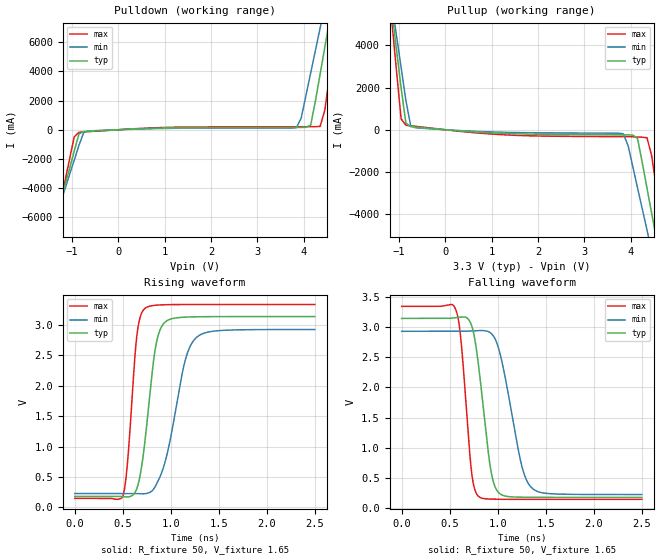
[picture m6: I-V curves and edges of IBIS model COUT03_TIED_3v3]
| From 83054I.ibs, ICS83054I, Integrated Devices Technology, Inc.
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[Model] COUT03_TIED_3v3
Model_type   Output
Polarity   Non-Inverting
|   typ   min   max
C_comp   2pF   1.5pF   2.5pF
Vmeas = 2.3V
Rref = 50
Vref = 1.65V
|   typ   min   max
[Voltage range]   3.3V   3.135V   3.465V
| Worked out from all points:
|   slope of the pulldown table from 0 to 0.495 V, typ, clamps not added: 6.88 ohm
|   slope of the pullup table from 0 to 0.495 V, typ, clamps not added: 5.83 ohm
|   rising waveform, R_fixture 50, V_fixture 1.65: 20-80 % time 127ps typ, 201ps min, 86.2ps max; typ from 0.181 V to 3.14 V
|   falling waveform, R_fixture 50, V_fixture 1.65: 20-80 % time 129ps typ, 191ps min, 93.3ps max; typ from 3.14 V to 0.181 V
[pulldown]
|Voltage   I (typ)   I (min)   I (max)
-3.3V     -29.26A    -25.24A    -35.98A
-1.463V   -7.508A    -7.113A    -8.217A
-1.361V   -6.298A    -6.106A    -6.67A
-952.6mV  -1.454A    -2.076A    -481.7mA
-850.5mV  -293.8mA   -1.069A    -175.5mA
-646.4mV  -102mA     -81.18mA   -129.6mA
3.844V    159mA      144.7mA    203.8mA
4.151V    319.9mA    3.884A     206.6mA
4.355V    3.815A     6.961A     228.9mA
4.559V    7.514A     10.04A     3.725A
4.763V    11.22A     13.12A     8.46A
6.6V      44.81A     41.05A     51.4A
[pullup]
|Voltage   I (typ)   I (min)   I (max)
-3.3V     44.73A     38.54A     55.09A
-1.157V   5.7A       6.046A     5.224A
-1.055V   3.84A      4.498A     2.846A
-952.6mV  1.979A     2.95A      516.9mA
-850.5mV  318.6mA    1.402A     214.1mA
-748.5mV  147.6mA    205.9mA    188.2mA
3.844V    -239.7mA   -193.2mA   -328.3mA
4.151V    -416.1mA   -2.755A    -342.5mA
4.355V    -2.772A    -4.758A    -379.9mA
4.559V    -5.183A    -6.764A    -2.792A
4.763V    -7.594A    -8.771A    -5.873A
6.6V      -29.3A     -26.85A    -33.6A
[Ramp]
|   typ   min   max
dV/dt_r   2.375/0.197n   2.163/0.318n   2.565/0.133n
dV/dt_f   2.386/0.194n   2.170/0.286n   2.577/0.141n
[Rising Waveform]
R_fixture = 50
V_fixture = 1.65
V_fixture_max = 1.73
V_fixture_min = 1.57
C_fixture = 0.0p
| Time   typ   min   max
0s        180.7mV    228.1mV    148.5mV
502ps     176mV      228.1mV    194.5mV
549.7ps   171.3mV    228.4mV    749mV
645.1ps   305mV      227.5mV    2.809V
730.4ps   1.085V     224.9mV    3.275V
823.3ps   2.449V     306.6mV    3.324V
888.5ps   2.925V     508.2mV    3.332V
1.147ns   3.131V     2.404V     3.339V
1.26ns    3.137V     2.786V     3.339V
2.5ns     3.141V     2.927V     3.339V
[Falling Waveform]
R_fixture = 50
V_fixture = 1.65
V_fixture_max = 1.73
V_fixture_min = 1.57
C_fixture = 0.0p
| Time   typ   min   max
0s        3.141V     2.927V     3.339V
562.2ps   3.152V     2.927V     3.29V
617.5ps   3.161V     2.927V     2.782V
727.9ps   3.024V     2.935V     602.1mV
803.2ps   2.328V     2.941V     193.8mV
926.2ps   652.8mV    2.9V       152.1mV
1.022ns   242.6mV    2.575V     149.5mV
1.242ns   183.7mV    755.2mV    148.5mV
1.353ns   181.7mV    341mV      148.5mV
2.5ns     180.7mV    228.1mV    148.5mV
